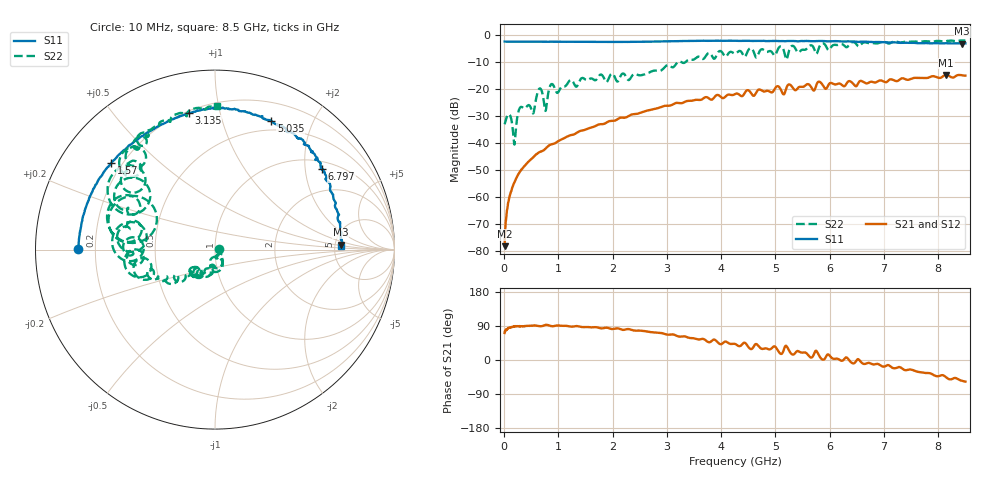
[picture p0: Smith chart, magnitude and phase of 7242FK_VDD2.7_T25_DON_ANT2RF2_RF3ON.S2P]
!Agilent Technologies,E5071C,MY46417908,A.11.23
!Date: Wed Dec 09 15:39:35 2020
!Data & Calibration Information:
!Freq	S11:SOLT2(ON)	S21:SOLT2(ON)	S12:SOLT2(ON)	S22:SOLT2(ON)
!PortZ  Port1:50+j0  Port2:50+j0
!Above PortZ is port z conversion or system Z0 setting when saving the data.
!When reading, reference impedance value at option line is always used.
# Hz S dB R 50
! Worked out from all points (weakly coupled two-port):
!   1601 points, 10 MHz to 8.5 GHz, reference 50 ohm
!   highest |S21| = -14.69 dB at 8.144 GHz (marker M1); lowest = -78.1 dB at 10 MHz (marker M2)
!   lowest |S11| = -3.1 dB at 8.442 GHz (marker M3), VSWR 5.68, Z = 281 + j30.1 ohm
!   |S11| at or under -10 dB: nowhere
!   |S22| runs from -40.5 to -1.9 dB; largest |S21 - S12| = 0.0027
!   S11 on the Smith chart (normalised r, x): 10 MHz: 0.13, +0.00; 1.57 GHz: 0.16, +0.35; 3.135 GHz: 0.21, +0.80; 5.035 GHz: 0.39, +1.46; 6.797 GHz: 1.22, +2.46; 8.5 GHz: 5.74, +0.46
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1e7  -2.34 179.7  -78.12 71.3  -77.12 74.2  -32.99 3.3
9.49e7  -2.38 177.4  -60.27 84.9  -60.33 85.6  -29.28 -43.2
1.904125e8  -2.39 174.8  -54.39 88.2  -54.47 88.5  -40.50 -45.3
3.177625e8  -2.41 171.4  -49.78 89.0  -49.88 89.1  -26.53 -55.6
5.353188e8  -2.41 165.8  -45.25 90.6  -45.29 91.0  -28.98 -70.4
6.520562e8  -2.41 162.8  -43.28 89.4  -43.31 89.4  -19.76 -80.1
7.634875e8  -2.42 160.2  -42.02 92.8  -42.03 92.7  -28.04 -86.9
8.696125e8  -2.41 157.4  -40.45 89.5  -40.44 89.4  -18.12 -84.1
1.426769e9  -2.45 143.9  -35.32 87.2  -35.32 87.1  -15.94 -107.7
1.570038e9  -2.47 140.3  -34.37 86.5  -34.38 86.6  -16.25 -116.5
2.843538e9  -2.33 107.0  -26.94 72.2  -26.95 72.2  -13.18 -139.9
3.135381e9  -2.21 100.9  -25.34 66.8  -25.35 66.8  -11.56 -141.1
4.255e9  -2.06 80.6  -21.81 42.4  -21.82 42.3  -6.84 -177.5
5.035019e9  -2.13 66.3  -18.88 27.4  -18.87 27.3  -5.67 174.9
5.671769e9  -2.23 53.7  -19.67 6.8  -19.61 6.6  -3.81 143.6
5.788506e9  -2.19 52.7  -17.27 15.8  -17.25 16.1  -5.39 158.4
5.905244e9  -2.20 49.8  -19.52 2.7  -19.45 2.7  -3.29 137.0
6.796694e9  -2.55 36.9  -17.35 -11.6  -17.37 -11.5  -2.96 127.5
7.088538e9  -2.74 32.4  -16.67 -13.9  -16.73 -14.0  -3.08 123.8
8.144481e9  -2.97 7.9  -14.69 -46.0  -14.73 -45.8  -2.22 101.5
8.441631e9  -3.09 2.2  -14.85 -55.3  -14.93 -55.4  -1.97 91.0
8.5e9  -3.04 1.6  -14.98 -57.1  -15.08 -56.9  -1.95 89.1
